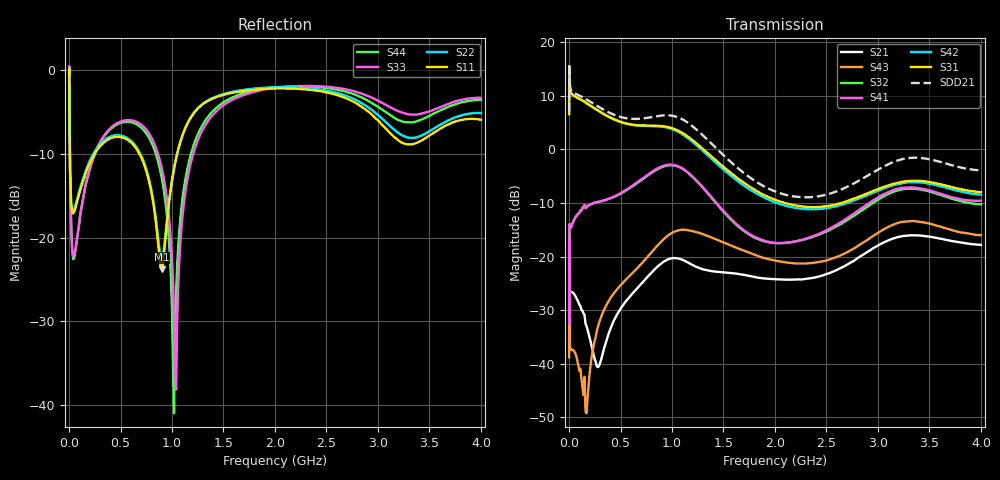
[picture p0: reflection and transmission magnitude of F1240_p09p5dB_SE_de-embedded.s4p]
! Integrated Device Technology
! Corporate Headquarters
! 6024 Silver Creek Valley Road
! San Jose, CA 95138  USA
! Phone:  1-408-284-8200
! Toll Free:  1-800-223-1366
! Webpage:  http://www.idt.com/
! Timing and RF Division
! 515 Groton Road, Suite 102
! Westford, MA 01886-6024
! Device:  F1240
! Description: Dual Intermediate Frequency Digital Variable Gain Amplifier
! Frequency:  10.0 -  500.00 MHz
! Package:  5x5 mm QFN Plastic Package: 32 pin
! Ports:  8 RF, 20 DC
!  Pin  1  = GA3 / Data  Pin 17  = RF OUT_B+
!  Pin  2  = GA4 / CLK  Pin 18  = RF OUT_B-
!  Pin  3  = GA5  Pin 19  = STBY_B
!  Pin  4  = VMODE  Pin 20  = Ground
!  Pin  5  = No Connect  Pin 21  = Ground
!  Pin  6  = GB5  Pin 22  = STB_A
!  Pin  7  = GB4  Pin 23  = RF OUT_A-  = Port 4
!  Pin  8  = GB3  Pin 24  = RF OUT_A+  = Port 3
!  Pin  9  = GB2  Pin 25  = GA0
!  Pin 10  = GB1  Pin 26  = ISET_A
!  Pin 11  = RF IN_B+  Pin 27  = VCC
!  Pin 12  = RF IN_B-  Pin 28  = Ground
!  Pin 13  = Ground  Pin 29  = RF IN_A-  = Port 2
!  Pin 14  = VCC  Pin 30  = RF IN_A+  = Port 1
!  Pin 15  = ISET_B  Pin 31  = GA1
!  Pin 16  = GB0  Pin 32  = GA2 / CSb
! Gain  = +19.5 dB
! State  = 1
! Voltage  = +5.00 V
! Current  = 85.292 mA (one channel only)
! Temperture  =  +25 C
! Test Date  =  2017-10-18
! Board  =  EB4031
! Data:  The device was measured on a custom evaluation board which has
!  individual transmission lines to the RF pins.  Data was collected
!  using a calibrated network analyzer.  The evaluation board was
!  de-embedded using Automatic Fixture Removal.
!  The reference plane is the edge of the package pin.
!  Only Channel A was measured.
!  This data is in single-ended operation.  If your needs are balanced
!  or differential S-parameters then this file needs to be used a
!  linear simulator.
! File Date:  2017-11-10  MJV
! Note:
!  Integrated Device Technology supplies this data as a sample of measured
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# Hz S dB R 100
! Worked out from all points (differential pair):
!   410 points, 500 kHz to 4 GHz, reference 100 ohm
!   strongest paths, dB at 500 kHz, 930 MHz, 1.96 GHz, 2.98 GHz, 4 GHz:
!     S31: 6.6, 4.3, -9.1, -7.5, -8.0
!     S42: 6.6, 4.2, -9.6, -7.9, -8.4
!     S41: -19.6, -3.0, -17.3, -9.2, -9.6
!     S32: -19.4, -3.1, -17.4, -9.6, -10.2
!     S43: -38.8, -16.6, -20.6, -15.8, -16.0
!     S21: -25.9, -20.8, -24.2, -18.2, -17.8
!   taken as a pair (ports 1,2 in; 3,4 out), SDD21 dB: 7.0, 6.4, -7.5, -4.0, -3.9
!   lowest |S11| = -23.8 dB at 900 MHz (marker M1), VSWR 1.14, Z = 111 + j7.74 ohm
!   |S11| at or under -10 dB: 8.092 MHz to 247.3 MHz (239.2 MHz wide, 187 % of centre); 684.5 MHz to 1.05 GHz (365.3 MHz wide, 42.1 % of centre)
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500000  -0.39 -5.7  -25.85 -4.0  -27.19 81.9  -58.58 69.8
        -25.86 -4.3  -0.39 -5.6  -58.45 69.6  -27.19 83.0
        6.62 -105.1  -19.38 61.8  -0.48 1.4  -38.85 -110.4
        -19.56 62.8  6.59 -104.0  -38.84 -110.1  -0.49 3.7
3000000  -2.83 -60.9  -28.26 -9.2  -16.03 24.2  -50.15 59.9
         -28.23 -8.7  -2.79 -60.8  -50.09 59.4  -16.03 24.4
         14.72 180.0  -17.59 6.9  -2.32 -56.5  -32.83 109.6
         -17.37 6.5  14.72 -179.8  -32.85 109.8  -2.38 -56.3
2e8  -11.12 -137.2  -35.08 -64.0  -18.02 -50.0  -34.44 15.7
     -35.16 -61.5  -10.85 -138.1  -34.41 16.4  -18.03 -50.1
     8.29 109.9  -10.35 -24.9  -11.84 -100.7  -43.09 119.4
     -10.34 -25.4  8.26 109.3  -41.79 107.3  -11.91 -99.5
5.3e8  -8.08 177.4  -29.57 -15.0  -19.11 -108.6  -28.66 -56.7
       -28.92 -17.1  -7.89 176.2  -28.77 -54.6  -19.24 -108.8
       4.99 26.4  -7.95 -88.8  -6.00 -159.0  -25.77 9.9
       -7.83 -90.3  4.93 25.5  -24.75 7.6  -6.19 -158.8
9e8  -23.79 32.4  -21.40 -85.9  -17.06 171.2  -25.39 -143.7
     -21.24 -92.5  -22.73 33.2  -25.62 -137.3  -17.35 170.5
     4.37 -66.5  -3.33 174.6  -11.66 136.8  -18.03 -69.5
     -3.18 170.7  4.26 -68.3  -17.11 -73.7  -12.86 138.2
1.21e9  -5.16 -113.1  -20.77 -171.3  -19.11 86.0  -25.40 142.4
        -21.69 -175.0  -5.09 -112.8  -25.03 149.5  -19.71 85.1
        1.57 -158.7  -5.32 66.5  -9.82 -100.3  -15.86 -163.4
        -5.27 61.7  1.26 -160.5  -15.30 -167.4  -8.94 -104.9
4e9  -5.90 -151.4  -17.92 79.3  -20.55 -63.5  -21.02 -48.0
     -17.82 78.7  -5.09 -148.3  -22.39 -28.5  -22.51 -56.2
     -7.98 19.4  -10.23 -98.5  -3.27 -139.3  -16.71 84.5
     -9.56 -112.3  -8.43 27.4  -16.01 59.9  -3.51 -146.3
